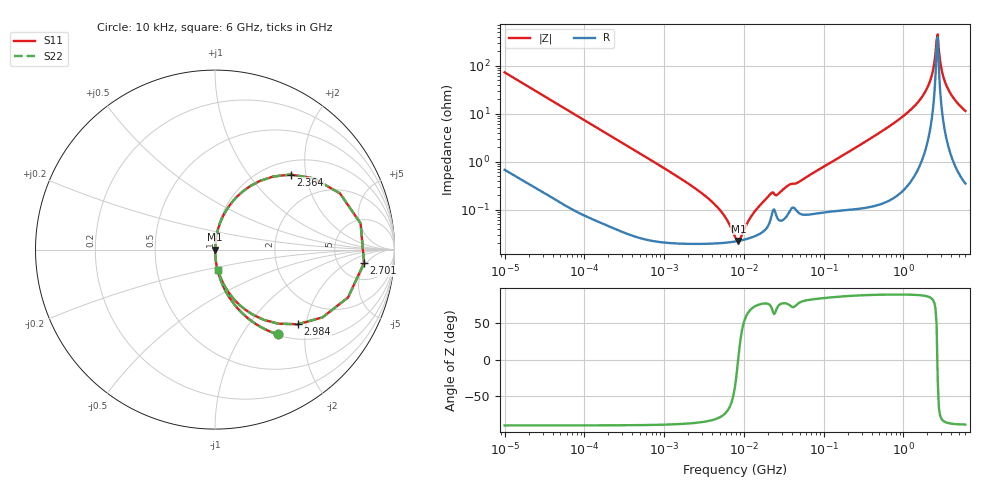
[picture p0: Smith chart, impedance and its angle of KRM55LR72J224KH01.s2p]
!Murata Part Number: KRM55LR72J224KH01
!These Parameters are Measured in Series Mode Connection
!Data Generated on Jan 08, 2026
!  o--ll--o
!Port1  Port2
!  o------o
!Operation Temp=25[degC], DC Bias Voltage=0[V]
!Freq. Start=10[kHz] Stop=6[GHz] 401[Steps]
# Hz S RI R 50
!Freq.(Hz) S11(Real) S11(Imag) S21(Real) S21(Imag) S12(Real) S12(Imag) S22(Real) S22(Imag)
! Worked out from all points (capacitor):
!   401 points, 10 kHz to 6 GHz, reference 50 ohm
!   read as one part in series: C = 217 nF near 10.69 kHz
!   lowest |Z| = 22.5 mohm at 8.559 MHz (marker M1)
!   series resonance near 8.494 MHz, so ESL is about 1.6 nH
!   S11 on the Smith chart (normalised r, x): 10 kHz: 1.01, -1.46; 2.364 GHz: 1.27, +1.64; 2.701 GHz: 8.89, -4.35; 2.984 GHz: 1.33, -1.80; 6 GHz: 1.01, -0.23
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10000  0.3499 -0.4723  0.6501 0.4723  0.6501 0.4723  0.3499 -0.4723
24549  0.0845 -0.2735  0.9155 0.2735  0.9155 0.2735  0.0845 -0.2735
92862  0.00711 -0.0791  0.9929 0.0791  0.9929 0.0791  0.00711 -0.0791
862344  0.000288 -0.00858  0.9997 0.00858  0.9997 0.00858  0.000288 -0.00858
4117309  0.0002 -0.00139  0.9998 0.00139  0.9998 0.00139  0.0002 -0.00139
5936256  0.000207 -0.000644  0.9998 0.000644  0.9998 0.000644  0.000207 -0.000644
7745967  0.000218 -0.000162  0.9998 0.000162  0.9998 0.000162  0.000218 -0.000162
8558778  0.000225 1.36e-05  0.9998 -1.36e-05  0.9998 -1.36e-05  0.000225 1.36e-05
1.275723e7  0.000269 0.000741  0.9997 -0.000741  0.9997 -0.000741  0.000269 0.000741
2.101053e7  0.000547 0.00196  0.9995 -0.00196  0.9995 -0.00196  0.000547 0.00196
2.651885e7  0.000659 0.00198  0.9993 -0.00198  0.9993 -0.00198  0.000659 0.00198
7.193098e7  0.000845 0.00564  0.9992 -0.00564  0.9992 -0.00564  0.000845 0.00564
6.67969e8  0.00457 0.0548  0.9954 -0.0548  0.9954 -0.0548  0.00457 0.0548
1.811831e9  0.0742 0.2363  0.9258 -0.2363  0.9258 -0.2363  0.0742 0.2363
2.139659e9  0.1958 0.3535  0.8042 -0.3535  0.8042 -0.3535  0.1958 0.3535
2.364181e9  0.4223 0.4181  0.5777 -0.4181  0.5777 -0.4181  0.4223 0.4181
2.526803e9  0.6963 0.3131  0.3037 -0.3131  0.3037 -0.3131  0.6963 0.3131
2.700612e9  0.8306 -0.0746  0.1694 0.0746  0.1694 0.0746  0.8306 -0.0746
2.983997e9  0.4623 -0.4159  0.5377 0.4159  0.5377 0.4159  0.4623 -0.4159
3.297118e9  0.2118 -0.3631  0.7882 0.3631  0.7882 0.3631  0.2118 -0.3631
3.643096e9  0.1117 -0.2834  0.8883 0.2834  0.8883 0.2834  0.1117 -0.2834
6e9  0.0163 -0.1123  0.9837 0.1123  0.9837 0.1123  0.0163 -0.1123
